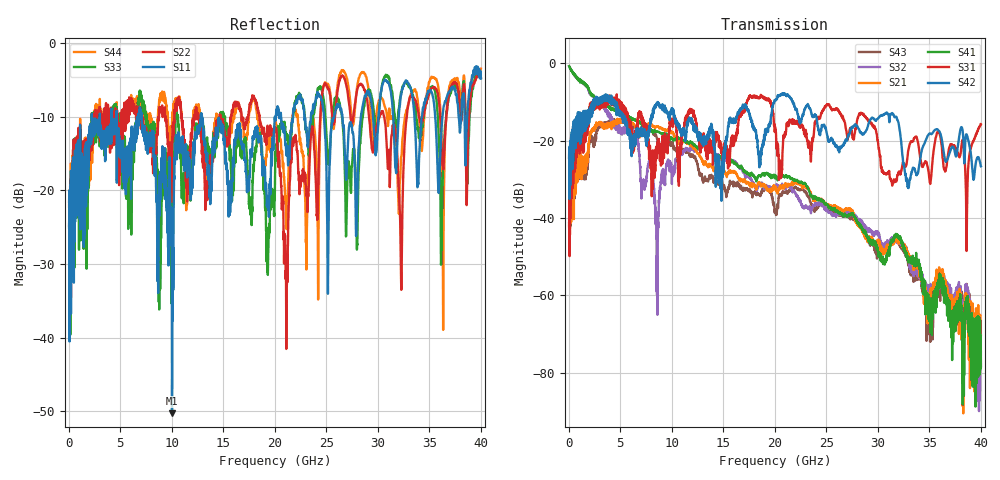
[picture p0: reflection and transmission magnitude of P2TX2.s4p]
!Agilent Technologies,N5245A,MY49151084,A.09.20.08
!Agilent N5245A: A.09.20.08
!Date: Thursday, March 01, 2012 10:34:34
!Correction: S11(Full 4 Port(1,2,3,4))
!S12(Full 4 Port(1,2,3,4))
!S13(Full 4 Port(1,2,3,4))
!S14(Full 4 Port(1,2,3,4))
!S21(Full 4 Port(1,2,3,4))
!S22(Full 4 Port(1,2,3,4))
!S23(Full 4 Port(1,2,3,4))
!S24(Full 4 Port(1,2,3,4))
!S31(Full 4 Port(1,2,3,4))
!S32(Full 4 Port(1,2,3,4))
!S33(Full 4 Port(1,2,3,4))
!S34(Full 4 Port(1,2,3,4))
!S41(Full 4 Port(1,2,3,4))
!S42(Full 4 Port(1,2,3,4))
!S43(Full 4 Port(1,2,3,4))
!S44(Full 4 Port(1,2,3,4))
!S4P File: Measurements: <S11,S12,S13,S14>,
!<S21,S22,S23,S24>,
!<S31,S32,S33,S34>,
!<S41,S42,S43,S44>:
# Hz S  dB  R 50
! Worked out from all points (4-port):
!   3996 points, 50 MHz to 40 GHz, reference 50 ohm
!   strongest paths, dB at 50 MHz, 10.04 GHz, 20.03 GHz, 30.02 GHz, 40 GHz:
!     S42: -24.3, -12.5, -9.6, -14.3, -26.6
!     S31: -24.5, -14.6, -16.4, -20.4, -15.7
!     S41: -0.7, -19.3, -29.1, -48.9, -78.4
!     S21: -42.0, -17.8, -31.9, -45.9, -70.4
!     S32: -0.7, -28.0, -32.3, -44.0, -74.6
!     S43: -41.3, -21.3, -38.4, -49.2, -78.3
!   lowest |S11| = -50.3 dB at 10.03 GHz (marker M1), VSWR 1.01, Z = 50.3 + j0.128 ohm
!   |S11| at or under -10 dB: start of sweep to 2.239 GHz; 7.076 GHz to 12.83 GHz (5.751 GHz wide, 57.8 % of centre); 12.9 GHz to 20.05 GHz (7.146 GHz wide, 43.4 % of centre)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
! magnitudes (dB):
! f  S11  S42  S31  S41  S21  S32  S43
! 50 MHz  -21.5  -24.3  -24.5  -0.7  -42.0  -0.7  -41.3
! 8.55 GHz  -20.8  -10.6  -24.6  -17.7  -16.4  -59.0  -19.2
! 10.03 GHz  -50.3  -12.5  -14.8  -19.5  -17.8  -29.4  -20.7
! 21.09 GHz  -14.2  -8.4  -17.8  -29.0  -31.1  -31.9  -33.1
! 24.84 GHz  -11.1  -16.2  -11.5  -36.5  -36.2  -37.9  -37.5
! 32.24 GHz  -7.1  -19.8  -28.2  -45.9  -46.3  -46.9  -47.8
! 40 GHz  -4.8  -26.6  -15.7  -78.4  -70.4  -74.6  -78.3
